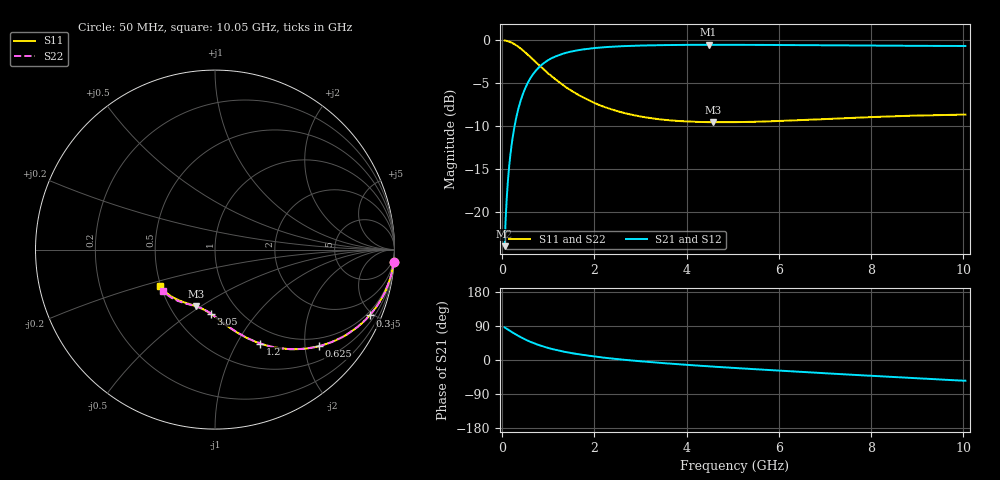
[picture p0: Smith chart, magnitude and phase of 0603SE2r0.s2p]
! AVX Thin Film Operation		Date: August 2001
! Description: Accu-P® Series, Thin Film, SMD, RF Capacitor
! Part Number: 06035J2R0ABT
! 50 MHz  -  10.05 GHz
! Serial Measurements
# mhz S db R 50
!	S11		S21		S12		S22
!	dB	Phase	dB	Phase	dB	Phase	dB	Phase
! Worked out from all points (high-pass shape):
!   401 points, 50 MHz to 10.05 GHz, reference 50 ohm
!   highest |S21| = -0.52 dB at 4.475 GHz (marker M1); lowest = -24.0 dB at 50 MHz (marker M2)
!   |S21| within 3 dB of the highest: 730 MHz to end of sweep
!   lowest |S11| = -9.6 dB at 4.575 GHz (marker M3), VSWR 2.00, Z = 33.7 - j24 ohm
!   |S11| at or under -10 dB: nowhere
!   |S22| runs from -9.5 to 0.0 dB; largest |S21 - S12| = 0
!   S11 on the Smith chart (normalised r, x): 50 MHz: 1, -29; 300 MHz: 0.80, -4.76; 625 MHz: 0.80, -2.31; 1.2 GHz: 0.80, -1.26; 3.05 GHz: 0.74, -0.61; 10.05 GHz: 0.49, -0.23
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50  -0.02 -4.0  -24.00 86.0  -24.00 86.0  -0.02 -4.0
75  -0.04 -6.0  -20.56 84.0  -20.56 84.0  -0.04 -6.0
125  -0.11 -10.0  -16.18 80.0  -16.18 80.0  -0.11 -10.0
175  -0.20 -13.8  -13.35 76.2  -13.35 76.2  -0.20 -13.8
225  -0.33 -17.6  -11.36 72.4  -11.36 72.4  -0.33 -17.6
300  -0.57 -23.1  -9.07 66.9  -9.07 66.9  -0.57 -23.1
375  -0.86 -28.2  -7.46 61.8  -7.46 61.8  -0.86 -28.2
450  -1.18 -33.0  -6.22 57.0  -6.22 57.0  -1.18 -33.0
625  -2.03 -42.8  -4.28 47.2  -4.28 47.2  -2.03 -42.7
900  -3.40 -54.8  -2.66 35.2  -2.66 35.2  -3.39 -54.8
1200  -4.72 -64.3  -1.79 25.7  -1.79 25.7  -4.72 -64.2
1425  -5.62 -70.1  -1.40 19.9  -1.40 19.9  -5.62 -70.0
1725  -6.58 -76.1  -1.08 13.9  -1.08 13.9  -6.58 -76.0
2300  -7.92 -85.2  -0.77 4.9  -0.77 4.9  -7.92 -84.9
3050  -8.93 -94.0  -0.60 -3.8  -0.60 -3.8  -8.92 -93.4
3400  -9.20 -97.6  -0.57 -7.4  -0.57 -7.4  -9.19 -96.8
4475  -9.55 -107.0  -0.52 -16.7  -0.52 -16.7  -9.53 -105.8
4575  -9.55 -108.2  -0.52 -17.5  -0.52 -17.5  -9.54 -106.6
5050  -9.54 -112.0  -0.53 -21.1  -0.53 -21.1  -9.53 -110.0
6725  -9.25 -124.0  -0.57 -33.0  -0.57 -33.0  -9.23 -121.0
8400  -8.88 -136.1  -0.63 -44.2  -0.63 -44.2  -8.85 -132.1
10050  -8.66 -146.8  -0.66 -54.7  -0.66 -54.7  -8.63 -141.8
